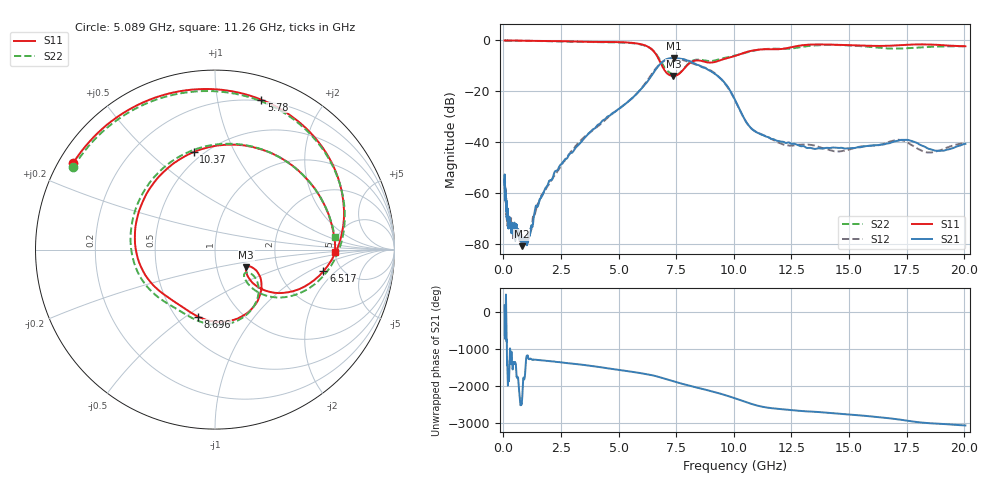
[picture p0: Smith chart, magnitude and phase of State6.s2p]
# Hz S DB R 50
!freq MagS11 AngS11 MagS21 AngS21 MagS12 AngS12 MagS22 AngS22
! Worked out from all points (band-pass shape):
!   1601 points, 50 MHz to 20.05 GHz, reference 50 ohm
!   highest |S21| = -6.86 dB at 7.402 GHz (marker M1); lowest = -81.0 dB at 793.7 MHz (marker M2)
!   |S21| within 3 dB of the highest: 6.744 GHz to 8.513 GHz (1.77 GHz wide, 23.2 % of centre)
!   lowest |S11| = -13.9 dB at 7.374 GHz (marker M3), VSWR 1.50, Z = 69.4 - j14.4 ohm
!   |S11| at or under -10 dB: 6.886 GHz to 7.953 GHz (1.067 GHz wide, 14.4 % of centre)
!   |S22| runs from -13.5 to 0.0 dB; largest |S21 - S12| = 0.025
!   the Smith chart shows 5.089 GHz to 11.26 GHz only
!   S11 on the Smith chart (normalised r, x): 5.089 GHz: 0.04, +0.28; 5.78 GHz: 0.19, +1.34; 6.517 GHz: 3.62, -1.41; 8.696 GHz: 0.64, -0.56; 10.37 GHz: 0.45, +0.70; 11.26 GHz: 5.05, -0.23
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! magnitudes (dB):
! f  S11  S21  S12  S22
! 50 MHz  0.0  -56.8  -55.6  0.0
! 135.9 MHz  0.0  -65.5  -67.5  0.0
! 145.4 MHz  0.0  -69.5  -68.8  0.0
! 178 MHz  0.0  -66.8  -72.5  0.0
! 369.6 MHz  0.0  -72.7  -72.4  0.0
! 423 MHz  0.0  -74.4  -76.7  0.0
! 521.7 MHz  -0.1  -77.1  -75.3  -0.1
! 560.2 MHz  -0.1  -72.5  -73.6  -0.1
! 793.7 MHz  -0.1  -81.0  -76.1  -0.1
! 1.005 GHz  -0.1  -80.3  -77.9  -0.1
! 2.722 GHz  -0.3  -46.6  -46.5  -0.4
! 5.089 GHz  -0.7  -26.4  -26.3  -0.8
! 5.78 GHz  -1.2  -21.0  -21.0  -1.3
! 6.517 GHz  -4.2  -12.7  -12.2  -4.1
! 7.374 GHz  -13.9  -6.9  -7.1  -13.4
! 7.402 GHz  -13.9  -6.9  -7.1  -13.4
! 8.696 GHz  -8.3  -10.6  -10.5  -7.8
! 9.585 GHz  -7.3  -16.5  -16.7  -6.9
! 10.37 GHz  -5.1  -29.4  -29.5  -5.1
! 11.26 GHz  -3.5  -37.2  -37.1  -3.5
! 14.47 GHz  -1.7  -42.2  -43.6  -1.8
! 20.05 GHz  -2.3  -40.7  -40.3  -2.3
